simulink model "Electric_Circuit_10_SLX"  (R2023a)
settings: Solver=ode23s  StartTime=0.0  StopTime=10.0  MaxStep=0.001  RelTol=1e-3
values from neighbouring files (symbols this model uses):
  C_6 = 0.001*F    (= 0.001)    [Electric_Circuit_10_EQN.m]    (also in Electric_Circuit_10_SLX_m.m; Electric_Circuit_01_EQN.m; Electric_Circuit_01_SLX_m.m; Electric_Circuit_03_EQN.m)
  C_7 = 0.001*F    (= 0.001)    [Electric_Circuit_10_EQN.m]    (also in Electric_Circuit_10_SLX_m.m; Electric_Circuit_02_EQN.m; Electric_Circuit_02_SLX_m.m; Electric_Circuit_04_EQN.m)
  I_3_0 = 0*A    (= 0)    [Electric_Circuit_10_SLX_m.m]    (also in Electric_Circuit_08_SLX_m.m; Inductive_Circuit_2_SLX_m.m)
  I_5_0 = 0*A    (= 0)    [Electric_Circuit_10_SLX_m.m]    (also in BIG_EC_Simscape_SLX_m.m; Electric_Circuit_01_SLX_m.m; Electric_Circuit_06_SLX_m.m; Electric_Circuit_09_SLX_m.m)
  I_9_0 = 0*A    (= 0)    [Electric_Circuit_10_SLX_m.m]    (also in BIG_EC_Simscape_SLX_m.m; Electric_Circuit_11_SLX_m.m)
  L_3 = 0.002*H    (= 0.002)    [Electric_Circuit_10_EQN.m]    (also in Electric_Circuit_10_SLX_m.m; Electric_Circuit_08_EQN.m; Electric_Circuit_08_SLX_m.m; Hydraulic_Circuit_01_EQN.m = 10)
  L_5 = 0.002*H    (= 0.002)    [Electric_Circuit_10_EQN.m]    (also in Electric_Circuit_10_SLX_m.m; BIG_EC_Simscape_EQN.m; BIG_EC_Simscape_SLX_m.m; Electric_Circuit_01_EQN.m)
  R_2 = 100*Ohm    (= 100)    [Electric_Circuit_10_EQN.m]    (also in Electric_Circuit_10_SLX_m.m; BIG_EC_Simscape_EQN.m; BIG_EC_Simscape_SLX_m.m; Electric_Circuit_07_EQN.m)
  R_4 = 100*Ohm    (= 100)    [Electric_Circuit_10_EQN.m]    (also in Electric_Circuit_10_SLX_m.m; BIG_EC_Simscape_EQN.m; BIG_EC_Simscape_SLX_m.m; Electric_Circuit_08_EQN.m)
  R_8 = 100*Ohm    (= 100)    [Electric_Circuit_10_EQN.m]    (also in Electric_Circuit_10_SLX_m.m; Hydraulic_Circuit_02_EQN.m = 10000; Hydraulic_Circuit_02_SLX_m.m = 10000)
  Ts = Tfin/Nr_Ts_Points    (= 0.0003)    [Electric_Circuit_10_SLX_m.m]    (also in BIG_EC_Simscape_SLX_m.m; Car_Dumper_SLX_m.m = 0.0022779; Electric_Circuit_01_SLX_m.m = 0.005; Electric_Circuit_02_SLX_m.m = 0.000480145)
  V_1_0 = 10*V    (= 10)    [Electric_Circuit_10_SLX_m.m]    (also in BIG_EC_Simscape_SLX_m.m; Electric_Circuit_02_SLX_m.m; Electric_Circuit_03_SLX_m.m; Electric_Circuit_04_SLX_m.m)
  V_6_0 = 0*V    (= 0)    [Electric_Circuit_10_SLX_m.m]    (also in Electric_Circuit_01_SLX_m.m; Electric_Circuit_03_SLX_m.m; Electric_Circuit_06_SLX_m.m; Electric_Circuit_08_SLX_m.m)
  V_7_0 = 0*V    (= 0)    [Electric_Circuit_10_SLX_m.m]    (also in Electric_Circuit_02_SLX_m.m; Electric_Circuit_04_SLX_m.m; Electric_Circuit_05_SLX_m.m; Electric_Circuit_07_SLX_m.m)

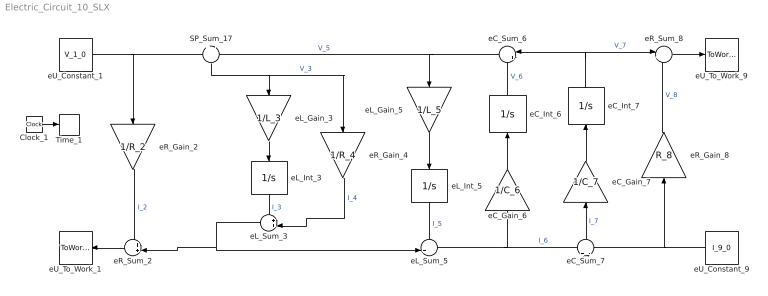
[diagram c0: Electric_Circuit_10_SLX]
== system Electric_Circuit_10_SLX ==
  Clock_1 : Clock
  SP_Sum_17 : Sum  Inputs=+|-
  Time_1 : ToWorkspace  VariableName=t  SaveFormat=Timeseries  SampleTime=Ts
  eC_Gain_6 : Gain  Gain=1/C_6  Multiplication=Matrix(K*u)
  eC_Gain_7 : Gain  Gain=1/C_7  Multiplication=Matrix(K*u)
  eC_Int_6 : Integrator  InitialCondition=V_6_0
  eC_Int_7 : Integrator  InitialCondition=V_7_0
  eC_Sum_6 : Sum  Inputs=|++
  eC_Sum_7 : Sum  Inputs=+|-
  eL_Gain_3 : Gain  Gain=1/L_3  Multiplication=Matrix(K*u)
  eL_Gain_5 : Gain  Gain=1/L_5  Multiplication=Matrix(K*u)
  eL_Int_3 : Integrator  InitialCondition=I_3_0
  eL_Int_5 : Integrator  InitialCondition=I_5_0
  eL_Sum_3 : Sum  Inputs=++|
  eL_Sum_5 : Sum  Inputs=-+|
  eR_Gain_2 : Gain  Gain=1/R_2  Multiplication=Matrix(K*u)
  eR_Gain_4 : Gain  Gain=1/R_4  Multiplication=Matrix(K*u)
  eR_Gain_8 : Gain  Gain=R_8  Multiplication=Matrix(K*u)
  eR_Sum_2 : Sum  Inputs=++|
  eR_Sum_8 : Sum  Inputs=|+-
  eU_Constant_1 : Constant  Value=V_1_0
  eU_Constant_9 : Constant  Value=I_9_0
  eU_To_Work_1 : ToWorkspace  VariableName=I_1_0  SaveFormat=Timeseries  SampleTime=Ts
  eU_To_Work_9 : ToWorkspace  VariableName=V_9_0  SaveFormat=Timeseries  SampleTime=Ts
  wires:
  eL_Sum_3/1 -> eR_Sum_2/2, eL_Sum_5/2
  eR_Sum_2/1 -> eU_To_Work_1/1
  eU_Constant_1/1 -> eR_Gain_2/1, SP_Sum_17/1
  eR_Gain_2/1 -> eR_Sum_2/1  "I_2"
  eC_Sum_6/1 -> SP_Sum_17/2, eL_Gain_5/1  "V_5"
  SP_Sum_17/1 -> eL_Gain_3/1, eR_Gain_4/1  "V_3"
  eR_Gain_4/1 -> eL_Sum_3/2  "I_4"
  eL_Gain_3/1 -> eL_Int_3/1
  eL_Int_3/1 -> eL_Sum_3/1  "I_3"
  eL_Sum_5/1 -> eC_Gain_6/1, eC_Sum_7/1  "I_6"
  eL_Gain_5/1 -> eL_Int_5/1
  eL_Int_5/1 -> eL_Sum_5/1  "I_5"
  eC_Int_7/1 -> eC_Sum_6/1, eR_Sum_8/1  "V_7"
  eC_Gain_6/1 -> eC_Int_6/1
  eC_Int_6/1 -> eC_Sum_6/2  "V_6"
  eU_Constant_9/1 -> eC_Sum_7/2, eR_Gain_8/1
  eC_Sum_7/1 -> eC_Gain_7/1  "I_7"
  eC_Gain_7/1 -> eC_Int_7/1
  eR_Sum_8/1 -> eU_To_Work_9/1
  eR_Gain_8/1 -> eR_Sum_8/2  "V_8"
  Clock_1/1 -> Time_1/1
